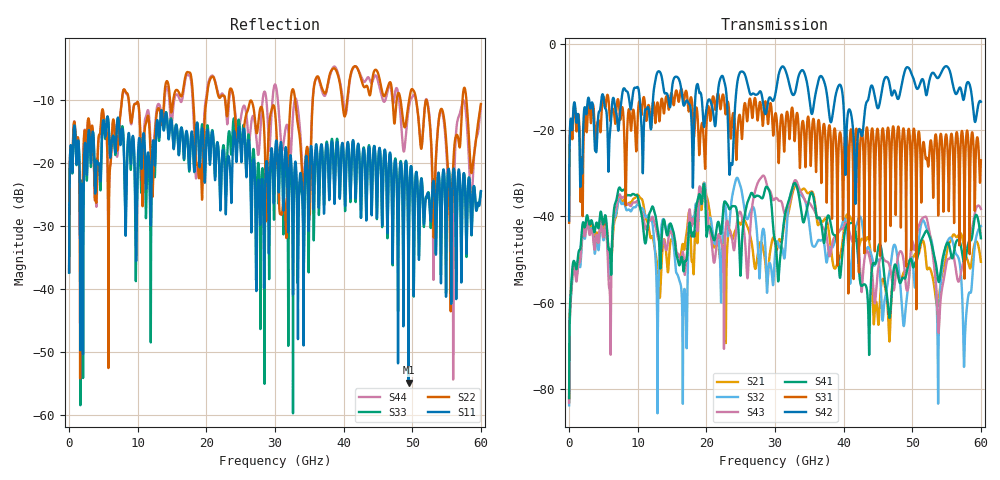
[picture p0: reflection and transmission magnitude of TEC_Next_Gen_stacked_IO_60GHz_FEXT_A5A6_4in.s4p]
!! CHANNEL DESCRIPTION:  Next Generation 28Gbps Press-fit Stacked I/O Connector
!!  with 4" 5-6-5 Megtron 6 Stripline trace on host side and 1.25" 7-5-7 Megtron 6 Microstrip trace on plug side
!! HOST PCB DESCRIPTION:  PCB thickness 3.425 mm
!!  26 Layer Board, 15 GND planes, 4 Layer route-out on Layers 7,11,17,21, 8mil stub on vias
!!  Pairs on following layers
!!  Layer 07 - A02A03 A14A15 D05D06
!!  Layer 11 - D020D3 C05C06 D14D15
!!  Layer 17 - C02C03 B05B06 C14C15
!!  Layer 21 - B02B03 A05A06 B14B15
!! CONNECTOR DESCRIPTION:  Next Generation 28Gbps Press-fit Stacked I/O Connector
!! PLUG-IN CARD DESCRIPTION:  PCB thickness 1mm thick
!!  6 Layer Board, 4 GND planes, 0.35 x 1.4mm mating pads
!!  Micro-strip diff traces referenced to GND plane 3mils down, 2nd GND plane 17mils from top of board
!!  PCB GND planes are symmetric
!! MODEL DESCRIPTION: TE Connectivity S-parameter model produced from Macro-model, Extracted .s4p FEXT (Victim B05B06 - Aggressor A05A06)
!! MODEL DATE: 5/15/2014 CR32f, FPR23
!! MODEL STATUS: Developmental
!! MODEL GEOMETRY: 4 Rows - Rows A, B, C, D. 3 pairs in each row, 12 total pairs
!! MODEL FREQUENCY RANGE: DC to 60 GHz in 10 MHz frequency steps
!! MODEL EDGE RATE LIMITATION: 8.33 ps (Using conservative 0.5/Fmax rule of thumb)
!! TIME-DOMAIN TRANSFORM CAUTIONS:
!! 1.) Do not simulate transient edge rates faster than the number listed above.  Edge
!!  rates faster than this number contain significant spectral content at frequencies
!!  above the model's highest frequency.
!! 2.) Even when simulating edge rates that are slower than the number listed above, be
!!  aware that the best time resolution possible with a direct iFFT is (1 / 2Fmax).
!!  As a result, time resolution is typically not adequate for most time-domain
!!  simulations unless tricks such as frequency-domain zero-padding and windowing are
!!  used to minimize leakage and aliasing.
!! 3.) Because the model has a uniform frequency step, a direct iFFT will result in an
!!  impulse that that has a time length given by either (1 / Fstep) or (1 / 2Fstep),
!!  depending on the transform being used.  Care has been taken in selecting the
!!  frequency step to ensure a settled impulse response for the model.  Therefore,
!!  convolution with the model's impulse response should present no issues.  However,
!!  if directly concatenating s-parameter models in the frequency domain a user must
!!  either interpolate necessary interim frequencies or complete impulse response
!!  zero-padding.  Impulse response zero-padding is more difficult, but more accurate.
!! PORT DEFINITIONS:
!! Port  1  ----->  Host A05		B05 Module <-----  Port  2
!! Port  3  ----->  Host A06		B06 Module <-----  Port  4
! Touchstone data
! Created: 29-Sep-2014 by IdEM R2011 (7.0.3)
# Hz S MA R 50
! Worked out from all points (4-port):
!   6000 points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, 10 MHz to 60 GHz, reference 50 ohm
!   strongest paths, dB at 10 MHz, 15.01 GHz, 30.01 GHz, 45.01 GHz, 60 GHz:
!     S42: -41.0, -10.1, -12.0, -14.9, -13.4
!     S31: -41.5, -11.8, -16.4, -20.1, -27.0
!     S41: -82.2, -42.5, -45.5, -47.4, -45.1
!     S43: -83.3, -44.1, -35.9, -52.5, -38.3
!     S32: -83.9, -44.5, -48.7, -50.1, -42.3
!     S21: -83.1, -45.4, -46.2, -64.3, -50.5
!   lowest |S11| = -54.9 dB at 49.46 GHz (marker M1), VSWR 1.00, Z = 49.8 - j0.0469 ohm
!   |S11| at or under -10 dB: start of sweep to end of sweep
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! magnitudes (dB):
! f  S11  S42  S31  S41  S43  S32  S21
! 10 MHz  -37.4  -41.0  -41.5  -82.2  -83.3  -83.9  -83.1
! 7.43 GHz  -16.7  -15.8  -17.2  -33.4  -35.0  -36.3  -35.8
! 16.85 GHz  -17.9  -14.0  -12.1  -50.7  -53.6  -57.1  -47.2
! 24.49 GHz  -18.0  -9.2  -22.6  -39.3  -41.1  -31.0  -42.2
! 49.46 GHz  -54.9  -5.5  -19.7  -51.0  -55.8  -55.6  -51.0
! 57.66 GHz  -23.2  -11.5  -35.3  -50.4  -49.3  -68.8  -48.1
! 60 GHz  -24.5  -13.4  -27.0  -45.1  -38.3  -42.3  -50.5
